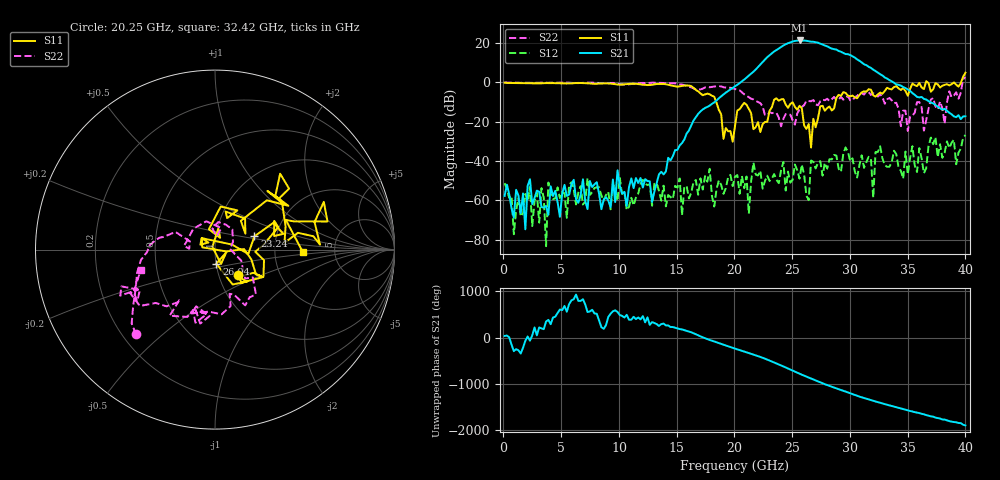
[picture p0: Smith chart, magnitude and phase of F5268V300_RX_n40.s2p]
!S2P File: Measurements: S11,S21,S12,S22
# MHz S  RI  R 50
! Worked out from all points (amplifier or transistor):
!   201 points, 100 MHz to 40 GHz, reference 50 ohm
!   highest |S21| = 21.2 dB at 25.64 GHz (marker M1)
!   |S21| within 3 dB of that: 24.12 GHz to 28.04 GHz (3.916 GHz wide, 15 % of centre)
!   unconditionally stable (mu >= 1): start of sweep to 36.54 GHz; 36.75 GHz to 39.66 GHz
!   at 6.684 GHz: K = 1250.55, MAG = -36.2 dB, |S12| = -52.9 dB
!   at 20.05 GHz: K = 88.35, MAG = 0.5 dB, |S12| = -48.1 dB
!   at 40 GHz: K = 131.86, MSG = 4.7 dB, |S12| = -26.8 dB
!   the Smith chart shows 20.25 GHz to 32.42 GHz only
!   S11 on the Smith chart (normalised r, x): 20.25 GHz: 1.24, -0.36; 23.24 GHz: 1.54, +0.24; 26.04 GHz: 1.00, -0.16; 32.42 GHz: 2.91, -0.11
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100  -0.9743 0.0392  0.00104 0.000759  -0.00111 0.00249  -0.9942 0.0366
6883  -0.4997 0.8025  -0.00112 0.00322  0.000643 -0.000434  0.0976 0.9546
13467  0.8487 0.3009  -0.00146 -0.0043  -0.00152 -0.00086  0.8868 -0.3601
20050  0.063 -0.0452  -0.4172 0.6696  -0.00174 -0.00353  -0.4142 -0.5255
20250  0.129 -0.1398  -0.2343 0.8267  -0.00257 0.00353  -0.4399 -0.4728
22045  -0.0736 0.0623  1.856 -1.58  0.00379 -0.00192  -0.3079 0.0663
23242  0.2196 0.0736  -5.026 -2.112  0.00341 -0.00106  -0.1555 0.0494
23841  0.3298 0.0756  -5.433 4.725  0.00192 0.00192  0.0351 0.1198
24439  0.2683 0.024  2.493 8.884  -0.000321 0.00173  0.0175 0.1539
25038  0.2698 -0.1523  10.74 1.444  0.000405 0.00325  0.1002 0.0431
25636  0.1777 -0.1785  5.773 -9.959  -0.00345 -0.000721  0.1588 -0.1247
26035  0.00773 -0.0786  -2.55 -11.13  0.00362 -0.00264  0.2101 -0.1545
26434  0.0336 -0.0798  -9.022 -6.21  -0.000501 -0.00087  0.2012 -0.2625
26833  0.0186 0.116  -10.58 1.313  0.00856 -0.00397  0.1682 -0.3106
27631  0.1245 0.2184  -0.3399 9.101  0.00219 -0.0036  0.0369 -0.3604
28429  0.1693 0.0886  6.813 2.157  0.0104 -0.00321  -0.0297 -0.37
29427  0.363 0.4229  1.866 -5.231  0.0126 -0.00877  -0.1228 -0.3372
30424  0.3932 0.1283  -3.948 -1.47  -0.0044 -0.00314  -0.2695 -0.3162
31422  0.5546 0.1534  -1.374 2.343  -0.00667 0.00648  -0.528 -0.2564
32419  0.4894 -0.0141  1.244 1.222  0.0097 0.0138  -0.4149 -0.1161
33417  0.5762 -0.3562  1.025 -0.4849  -0.0034 -0.00621  -0.3955 0.0468
40000  0.9465 -1.459  -0.0214 -0.1345  -0.0442 -0.0116  0.2975 -1.309
